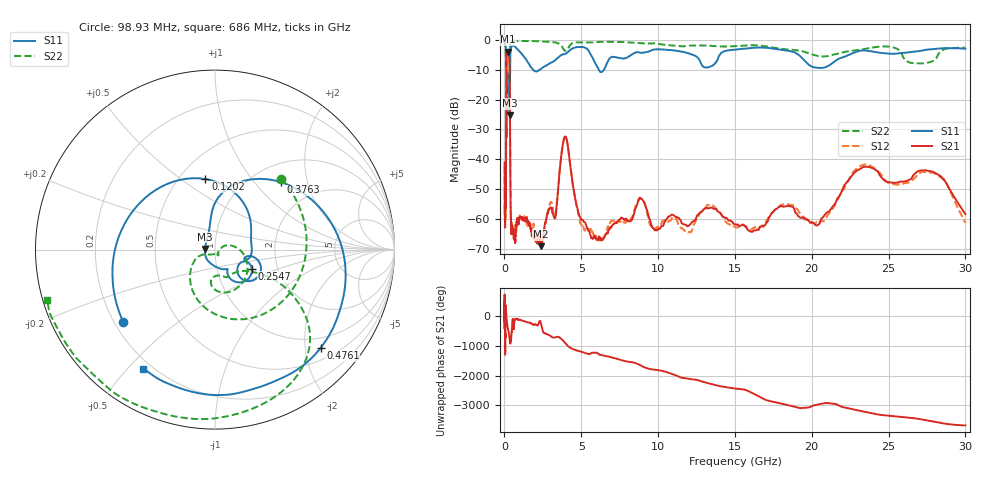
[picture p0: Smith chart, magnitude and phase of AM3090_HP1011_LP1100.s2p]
! Date/Time: Thu, Feb 28, 2019 2:06 PM
! Network Analyzer: Agilent Technologies E8364B Rev: A.07.50.67
! Sweep from 0.010 to 30.000 GHz, 1601 Points, Sweep Type: LOG
! Power Supply: 5.022 V, 0.002 A
# Hz S DB R 50
!freq MagS11 AngS11 MagS21 AngS21 MagS12 AngS12 MagS22 AngS22
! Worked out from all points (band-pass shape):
!   1601 points, 10 MHz to 30 GHz, reference 50 ohm
!   highest |S21| = -3.91 dB at 229.3 MHz (marker M1); lowest = -69.2 dB at 2.361 GHz (marker M2)
!   |S21| within 3 dB of the highest: 132.3 MHz to 324.1 MHz (191.8 MHz wide, 84.1 % of centre)
!   lowest |S11| = -25.2 dB at 333.7 MHz (marker M3), VSWR 1.12, Z = 44.8 + j0.343 ohm
!   |S11| at or under -10 dB: 124.5 MHz to 361.2 MHz (236.7 MHz wide, 97.4 % of centre); 1.864 GHz to 2.254 GHz (389.2 MHz wide, 18.9 % of centre); 6.144 GHz to 6.465 GHz (321.2 MHz wide, 5.09 % of centre)
!   |S22| runs from -32.8 to -0.1 dB; largest |S21 - S12| = 0.013
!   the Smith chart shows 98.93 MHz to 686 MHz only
!   S11 on the Smith chart (normalised r, x): 98.93 MHz: 0.23, -0.33; 120.2 MHz: 0.67, +0.62; 254.7 MHz: 1.47, -0.33; 376.3 MHz: 1.33, +1.38; 476.1 MHz: 0.75, -2.33; 686 MHz: 0.17, -0.55
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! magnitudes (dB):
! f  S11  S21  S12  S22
! 10 MHz  -0.3  -41.0  -42.3  -0.7
! 38.04 MHz  -0.4  -59.7  -60.2  -1.5
! 98.93 MHz  -3.7  -49.2  -46.3  -5.3
! 120.2 MHz  -8.0  -15.4  -15.5  -9.0
! 144.7 MHz  -13.9  -5.1  -5.0  -30.2
! 229.3 MHz  -16.1  -3.9  -3.9  -15.6
! 254.7 MHz  -12.7  -4.1  -4.0  -16.6
! 333.7 MHz  -25.2  -8.7  -8.6  -9.7
! 376.3 MHz  -5.6  -39.5  -39.6  -1.2
! 413.9 MHz  -2.9  -58.9  -59.8  -0.5
! 476.1 MHz  -1.9  -63.5  -62.0  -0.3
! 550.5 MHz  -1.9  -64.0  -65.8  -0.2
! 686 MHz  -2.2  -67.7  -63.7  -0.2
! 2.084 GHz  -10.5  -66.6  -66.5  -0.4
! 2.361 GHz  -9.8  -69.2  -67.9  -0.4
! 3.302 GHz  -6.7  -59.7  -59.0  -0.8
! 3.934 GHz  -4.6  -32.4  -32.3  -3.6
! 5.103 GHz  -2.4  -60.4  -62.4  -0.8
! 7.926 GHz  -6.0  -59.9  -61.0  -0.7
! 20.31 GHz  -9.2  -62.3  -61.1  -5.2
! 23.48 GHz  -3.5  -42.5  -41.8  -2.9
! 30 GHz  -2.9  -58.4  -61.3  -2.6
